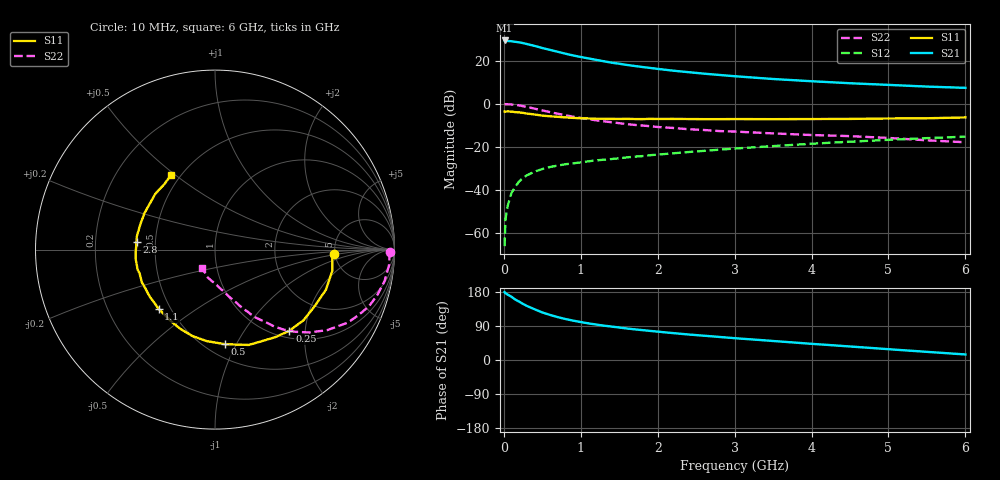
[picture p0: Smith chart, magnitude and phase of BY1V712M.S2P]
! SIEMENS Small Signal Semiconductors
! BFY420
! Si NPN RF SIEGET Grounded Emitter Transistor in MICRO-X
! VCE = 1.75 V  IC = 12 mA
! Common Emitter S-Parameters:  October  1996
# GHz  S  MA  R  50
!  f  S11  S21  S12  S22
! GHz  MAG  ANG  MAG  ANG  MAG  ANG  MAG  ANG
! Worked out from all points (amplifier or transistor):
!   36 points, 10 MHz to 6 GHz, reference 50 ohm
!   highest |S21| = 29.3 dB at 10 MHz (marker M1)
!   |S21| within 3 dB of that: start of sweep to 448.8 MHz
!   unconditionally stable (mu >= 1): 2.339 GHz to end of sweep
!   at 250 MHz: K = 0.22, MSG = 31.3 dB, |S12| = -34.4 dB
!   at 1.4 GHz: K = 0.81, MSG = 22.3 dB, |S12| = -25.6 dB
!   at 6 GHz: K = 1.09, MAG = 9.5 dB, |S12| = -15.3 dB
!   S11 on the Smith chart (normalised r, x): 10 MHz: 4.87, -0.44; 250 MHz: 1.14, -1.65; 500 MHz: 0.62, -0.90; 1.1 GHz: 0.43, -0.36; 2.8 GHz: 0.39, +0.04; 6 GHz: 0.45, +0.48
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0.01  0.6618 -2.2  29.3 179.2  0.0005 96.0  0.9728 -0.7
0.02  0.6553 -4.1  28.98 176.4  0.002 95.0  0.9727 -1.8
0.1  0.6571 -19.9  28.12 166.7  0.0086 82.2  0.9611 -10.5
0.15  0.639 -29.3  27.24 159.3  0.012 75.9  0.939 -15.7
0.2  0.6311 -38.6  26.48 154.0  0.0159 74.4  0.9137 -20.3
0.25  0.6133 -47.5  25.43 147.9  0.019 68.9  0.8766 -24.8
0.3  0.592 -55.6  24.23 142.6  0.022 66.7  0.8443 -28.8
0.4  0.5639 -70.4  21.91 133.9  0.0267 61.4  0.7703 -35.6
0.5  0.5302 -83.9  19.57 125.4  0.0307 58.2  0.7009 -41.2
0.6  0.512 -95.1  17.71 119.0  0.0342 55.5  0.6399 -45.7
0.7  0.4975 -104.8  16.02 113.2  0.0369 53.4  0.5873 -49.4
0.8  0.4821 -113.6  14.46 108.2  0.0396 51.7  0.5405 -52.4
0.9  0.47 -120.4  13.18 103.9  0.0416 50.6  0.501 -54.6
1.1  0.4555 -133.6  11.24 96.7  0.0464 50.2  0.4396 -59.2
1.3  0.4483 -143.8  9.653 90.7  0.0505 49.7  0.391 -62.2
1.6  0.4462 -155.9  7.932 83.1  0.0571 49.3  0.3376 -66.6
2.2  0.445 -173.0  5.844 71.0  0.071 48.6  0.2747 -73.3
2.8  0.4396 174.2  4.649 60.9  0.0861 46.7  0.2327 -79.1
3.5  0.4393 161.1  3.747 50.2  0.1044 43.2  0.2054 -85.4
4.5  0.4448 144.6  2.986 35.7  0.1318 36.3  0.1776 -95.1
5.5  0.4607 128.0  2.499 21.5  0.1597 27.7  0.1421 -112.4
6  0.482 120.6  2.336 14.6  0.1727 23.2  0.1279 -125.0
